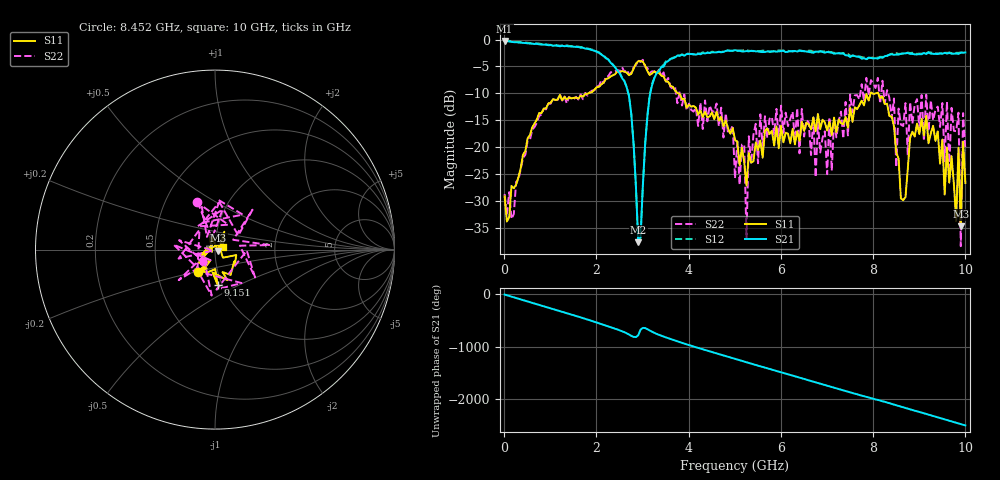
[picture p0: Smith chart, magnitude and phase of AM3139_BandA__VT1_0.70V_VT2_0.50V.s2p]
! Date/Time: Tue, Nov 13, 2018 4:56 PM
! Network Analyzer: Agilent Technologies E8364B Rev: A.07.50.67
! Sweep from 0.010 to 10.000 GHz, 201 Points, Sweep Type: LIN
! Power Supply: 0.700 V, 0.000 A
# Hz S DB R 50
!freq MagS11 AngS11 MagS21 AngS21 MagS12 AngS12 MagS22 AngS22
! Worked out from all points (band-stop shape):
!   201 points, 10 MHz to 10 GHz, reference 50 ohm
!   highest |S21| = -0.25 dB at 10 MHz (marker M1); lowest = -37.7 dB at 2.907 GHz (marker M2)
!   |S21| within 3 dB of the highest: start of sweep to 2.178 GHz; 3.717 GHz to 7.502 GHz (3.785 GHz wide, 67.5 % of centre)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
!   lowest |S11| = -34.7 dB at 9.9 GHz (marker M3), VSWR 1.04, Z = 51.8 - j0.536 ohm
!   |S11| at or under -10 dB: start of sweep to 1.824 GHz; 3.772 GHz to 7.947 GHz (4.174 GHz wide, 71.2 % of centre); 8.107 GHz to end of sweep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
!   |S22| runs from -38.4 to -3.8 dB; largest |S21 - S12| = 0.029
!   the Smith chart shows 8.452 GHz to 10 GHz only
!   S11 on the Smith chart (normalised r, x): 8.452 GHz: 0.80, -0.20; 9.151 GHz: 0.95, -0.39; 10 GHz: 1.09, +0.03
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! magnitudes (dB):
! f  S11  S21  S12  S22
! 10 MHz  -29.2  -0.2  -0.2  -28.7
! 1.708 GHz  -10.6  -1.5  -1.4  -11.1
! 2.657 GHz  -6.2  -8.9  -8.9  -5.6
! 2.907 GHz  -4.0  -37.7  -37.3  -3.9
! 3.357 GHz  -6.2  -5.9  -5.8  -5.6
! 5.005 GHz  -18.6  -2.0  -2.1  -25.8
! 5.205 GHz  -22.8  -2.2  -2.0  -19.5
! 5.255 GHz  -27.1  -2.1  -1.9  -37.1
! 5.305 GHz  -21.1  -2.2  -2.1  -18.0
! 5.554 GHz  -18.8  -2.3  -2.1  -13.9
! 6.703 GHz  -14.5  -2.5  -2.3  -14.5
! 6.753 GHz  -17.1  -2.3  -2.3  -25.6
! 8.352 GHz  -14.2  -2.8  -2.8  -10.8
! 8.452 GHz  -16.2  -2.8  -2.7  -11.0
! 8.501 GHz  -21.0  -2.8  -2.5  -23.7
! 8.651 GHz  -29.9  -2.6  -2.6  -16.1
! 9.151 GHz  -14.2  -2.7  -2.6  -10.3
! 9.8 GHz  -33.6  -2.6  -2.5  -17.0
! 9.85 GHz  -20.1  -2.7  -2.5  -13.6
! 9.9 GHz  -34.7  -2.5  -2.4  -38.4
! 9.95 GHz  -19.0  -2.5  -2.4  -13.7
! 10 GHz  -26.7  -2.4  -2.3  -20.6
